TYPE E_DriverHomeStep :
(
	STATE_DRIVERHOME_STANDSTILL		:= 10,	(* 待命 *) 
	STATE_DRIVERHOME_CLEARFLAG		:= 15,	(* 清除回零标志 *) 
	STATE_DRIVERHOME_DISABLELAG		:= 20,	(* 禁用误差监控 *) 
	STATE_DRIVERHOME_READSCLFCTR	:= 30,	(* 读比例因子 *) 
	STATE_DRIVERHOME_MODEHOME		:= 40,	(* 切换到回零模式 *) 
	STATE_DRIVERHOME_WRITEPARA1		:= 50,	(* 写入回零参数1 *) 
	STATE_DRIVERHOME_WRITEPARA2		:= 60,	(* 写入回零参数2 *) 
	STATE_DRIVERHOME_STARTHOME		:= 70,	(* 启动回零 *) 
	STATE_DRIVERHOME_CHECKSTATUS1	:= 80,	(* 等待完成 *) 
	STATE_DRIVERHOME_CHECKSTATUS2	:= 90,	(* 检查完成信号 *) 
	STATE_DRIVERHOME_RESETSETPOINT	:= 100,	(* 复位CSP设定值 *) 
	STATE_DRIVERHOME_MODECSP		:= 110,	(* 切换到CSP *) 
	STATE_DRIVERHOME_READPOSITION	:= 120,	(* 读驱动器反馈位置 *) 
	STATE_DRIVERHOME_CLEARPOS		:= 130,	(* 清除NC位置 *) 
	STATE_DRIVERHOME_ENABLELAG		:= 140,	(* 使能误差监控 *) 
	STATE_DRIVERHOME_SET_FLAG		:= 145,	(* 设置回零标志 *)
	
	STATE_DRIVERHOME_STOP1			:= 150,	(* 停止回零 *) 
	
	STATE_DRIVERHOME_ERRORSTOP		:= 800,	(* 驱动器回零错误停止 *) 
	STATE_DRIVERHOME_ERROR			:= 900,	(* 驱动器回零错误 *) 
	STATE_DRIVERHOME_STOP2			:= 960,	(* 停止回零 *) 
	STATE_DRIVERHOME_STOP3			:= 970,	(* 停止回零 *)
	STATE_DRIVERHOME_STOP4			:= 980,	(* 停止回零 *) 
	STATE_DRIVERHOME_STOP5			:= 990,	(* 停止回零 *)
	
	STATE_DRIVERHOME_DONE			:= 999	(* 驱动器回零完成 *) 
	
	
	
);
END_TYPE
